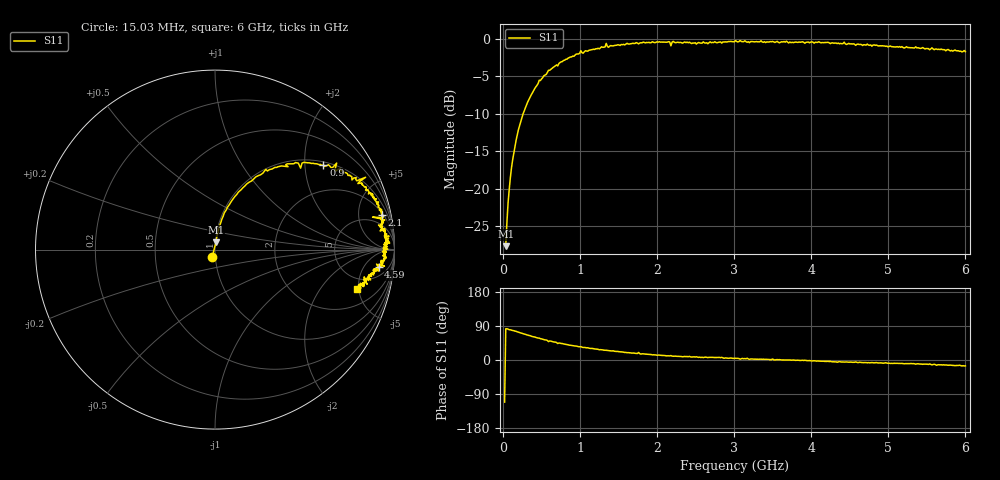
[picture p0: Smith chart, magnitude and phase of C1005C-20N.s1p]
!	Network	Analyzer	HP8753E.07.74:	Oct	30	2002	Serial	No.	JP38451487
!	Hewlett-Packard
!	7	Sep	2009	8:52:36
!	Frequency	S11
#	HZ	S	RI	R	50
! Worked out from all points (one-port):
!   400 points, 15.03 MHz to 6 GHz, reference 50 ohm
!   lowest |S11| = -27.6 dB at 30.03 MHz (marker M1), VSWR 1.09, Z = 50.4 + j4.15 ohm
!   |S11| at or under -10 dB: start of sweep to 255.1 MHz
!   S11 on the Smith chart (normalised r, x): 15.03 MHz: 0.97, -0.08; 900 MHz: 1.09, +2.49; 2.1 GHz: 2.42, +9.20; 4.59 GHz: 9, -11; 6 GHz: 3.56, -4.74
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1.502992e7  -0.0154 -0.0397
3.002985e7  0.00544 0.0411
6.00297e7  0.012 0.0797
1.050295e8  0.0269 0.136
1.650292e8  0.052 0.205
2.550287e8  0.111 0.296
4.650277e8  0.283 0.447
7.650262e8  0.512 0.484
9.000255e8  0.604 0.471
1.320023e9  0.794 0.385
1.335023e9  0.839 0.403
1.365023e9  0.796 0.368
1.515022e9  0.839 0.331
1.740021e9  0.893 0.276
1.755021e9  0.869 0.314
1.785021e9  0.905 0.253
2.10002e9  0.929 0.191
2.160019e9  0.934 0.178
2.175019e9  0.878 0.181
2.205019e9  0.946 0.165
2.265019e9  0.935 0.16
2.505017e9  0.911 0.137
3.015015e9  0.97 0.0746
3.765011e9  0.942 0.000152
4.515007e9  0.92 -0.0887
4.590007e9  0.912 -0.0969
5.265004e9  0.861 -0.145
6e9  0.789 -0.219
